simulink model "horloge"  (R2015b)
settings: Solver=FixedStepDiscrete  StartTime=0.0  StopTime=inf  FixedStep=0.05  RelTol=1e-3

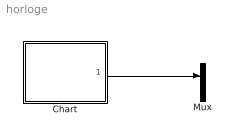
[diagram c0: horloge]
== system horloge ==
  Chart : Stateflow chart  TreatAsAtomicUnit=on
  Mux : Mux  Inputs=2
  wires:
  Chart/1(horl) -> Mux/1

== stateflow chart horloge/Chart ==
  state zero
    entry:horl;
  state un
    entry:horl;
  zero -> un : after(0.1,sec)
  (default) -> zero
  un -> zero : after(0.1,sec)
  events: output EITHER_EDGE_EVENT
